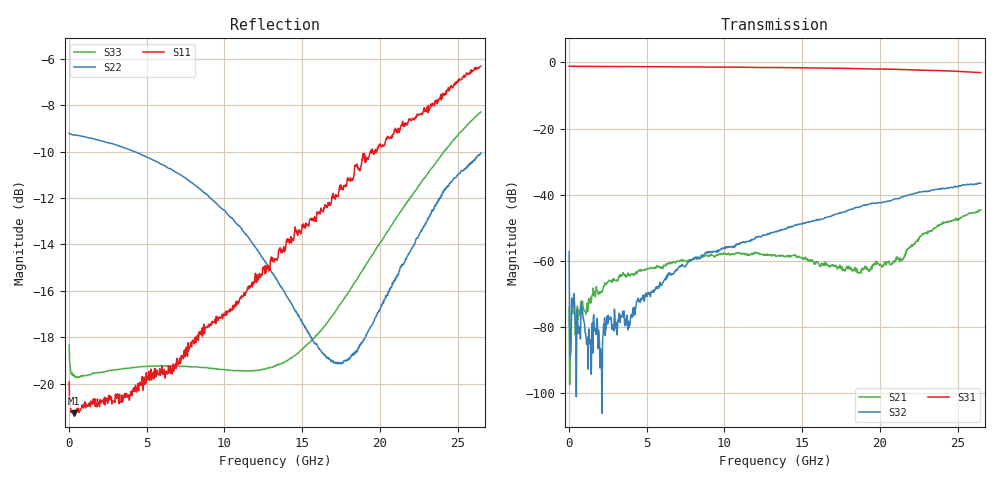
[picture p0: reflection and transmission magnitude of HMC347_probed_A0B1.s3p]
! Hittite Microwave Corporation
! 20 Alpha Road
! Chelmsford, MA 01824
! http://www.hittite.com
! Tel: 978-250-3343
! Fax: 978-250-3373
! Device:  HMC347
! Description: GaAs MMIC SPDT Non-Reflective Switch
! Frequency:  DC -  20.00 GHz
! Package:  DIE
! Ports:  3 RF, 2 DC
!  Pad  1 = RF1 = Port 2
!  Pad  2 = Control A [Alternate]
!  Pad  3 = Control B [Alternate]
!  Pad  4 = RFC = Port 1
!  Pad  5 = Control A [Alternate]
!  Pad  6 = Control B [Alternate]
!  Pad  7 = RF2 = Port 3
!  Pad  8 = Control A
!  Pad  9 = Control B
!  Pad 10 = Control A [Alternate]
! Control:  -5 Volt control voltage
!  Low  = 0 =  0 V
!  High = 1 = -5 V
! State:  RF2 Selected
! Voltages:  VA =  0.0 Volts
!  VB = -5.0 Volts
! Data:  The device was measured using G-S-G Probes at the chip ports.
!  Data was collected using an calibrated 3 port network analyzer.
!  The reference plane is the pads on the switch chip.
! Misc:  Die 64601
!  Lot GB01, Tested Unit 3
! Date Measured:  2010-03-11
! Date:  2010-03-15
! Note:
!  Hittite supplies this data as a sample of measured data at the package pin for
!  for this package product.  Your particular data for this product may vary.
!  Data was taken at 25 degrees C.
!  Hittite reserves the right to change this data at anytime.
!S3P File: Measurements: <S11,S12,S13>,
!  <S21,S22,S23>,
!  <S31,S32,S33>:
# Hz S  dB  R 50
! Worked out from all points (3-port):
!   801 points, 10 MHz to 26.5 GHz, reference 50 ohm
!   strongest paths, dB at 10 MHz, 6.633 GHz, 13.26 GHz, 19.88 GHz, 26.5 GHz:
!     S31: -1.1, -1.3, -1.6, -2.0, -3.1
!     S32: -57.1, -63.9, -51.2, -42.4, -36.5
!     S21: -74.0, -60.7, -58.1, -60.8, -44.5
!   lowest |S11| = -21.3 dB at 308 MHz (marker M1), VSWR 1.19, Z = 59.4 - j0.0625 ohm
!   |S11| at or under -10 dB: start of sweep to 19.39 GHz; 19.46384 GHz to 19.4916 GHz (27.76 MHz wide, 0.143 % of centre); 19.58 GHz to 19.69 GHz (106.5 MHz wide, 0.543 % of centre)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
1e7  -19.93 -0.3  -79.72 48.1  -1.10 -0.2
     -73.99 -2.4  -9.20 180.0  -72.25 -157.5
     -1.12 -0.1  -57.15 -88.7  -18.34 -0.9
1.755625e8  -21.17 -0.9  -71.63 112.5  -1.14 -1.2
            -71.13 109.8  -9.25 178.8  -71.29 111.3
            -1.15 -1.2  -72.45 109.0  -19.62 -2.2
3.080125e8  -21.28 -0.3  -70.48 60.9  -1.15 -2.0
            -71.35 66.6  -9.27 177.8  -70.02 63.4
            -1.16 -2.1  -69.83 63.3  -19.67 -2.9
1.168938e9  -20.97 -2.0  -74.08 59.5  -1.18 -7.4
            -72.75 63.5  -9.38 171.9  -88.90 -7.2
            -1.19 -7.4  -84.78 14.2  -19.63 -8.3
3.784825e9  -20.59 -9.0  -64.39 58.4  -1.24 -23.4
            -63.71 61.1  -9.88 155.1  -83.21 44.9
            -1.25 -23.5  -80.83 52.9  -19.34 -28.5
4.745088e9  -20.29 -10.3  -63.01 58.3  -1.24 -29.3
            -62.79 59.0  -10.15 149.0  -70.62 91.2
            -1.27 -29.3  -70.50 90.3  -19.26 -35.4
7.857662e9  -18.32 -19.0  -59.99 56.6  -1.33 -48.4
            -59.55 54.2  -11.33 128.0  -59.65 66.5
            -1.35 -48.4  -59.67 68.8  -19.28 -54.6
1.3255e10  -14.60 -34.5  -58.87 29.4  -1.55 -81.9
           -58.10 29.0  -15.37 78.4  -51.17 2.1
           -1.55 -82.0  -51.16 1.5  -19.23 -67.2
1.868545e10  -10.74 -50.2  -64.11 -64.7  -1.84 -117.1
             -63.49 -72.9  -18.34 -29.8  -43.83 -59.7
             -1.87 -117.1  -43.65 -59.8  -15.30 -66.5
2.65e10  -6.31 -77.9  -44.39 137.8  -2.98 -170.5
         -44.53 135.9  -10.05 -135.5  -37.04 -163.0
         -3.08 -170.9  -36.52 -163.5  -8.29 -102.4
